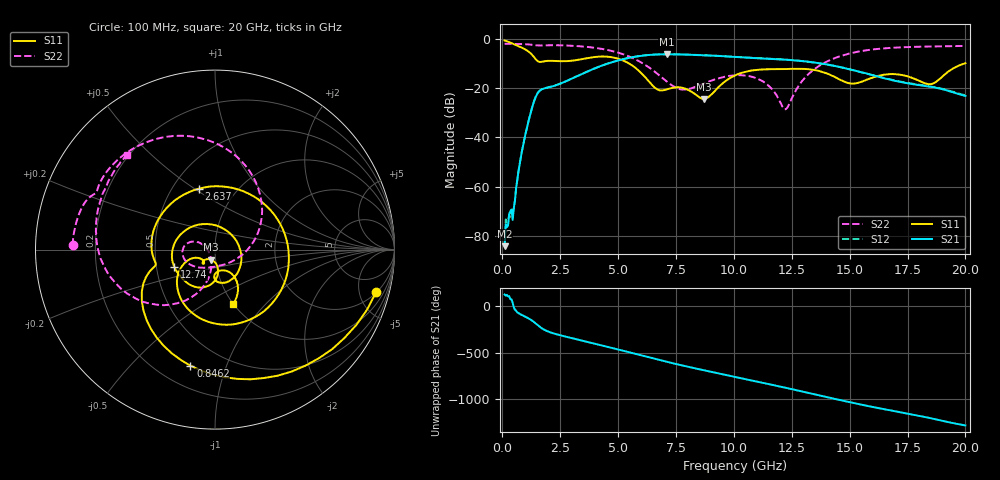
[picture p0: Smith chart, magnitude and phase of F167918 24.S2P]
!  2-Port S-parameters saved by WinCal
! VAR MeasName=S-Parameters (CALIBRATED_DATA) read from VNA (N5242A)
! VAR MeasDate=2016-11-22 10:25:54
! VAR NAME=F167918 24
! VAR FILENAME=F167918 24.S2P
! VAR DATE=2016-11-22 10:25:54
! VAR PHYS_PORTS=1,2
# Hz S DB R 50
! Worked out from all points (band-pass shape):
!   401 points, 100 MHz to 20 GHz, reference 50 ohm
!   highest |S21| = -6.24 dB at 7.115 GHz (marker M1); lowest = -84.2 dB at 100 MHz (marker M2)
!   |S21| within 3 dB of the highest: 4.827 GHz to 13.19 GHz (8.367 GHz wide, 92.9 % of centre)
!   lowest |S11| = -24.4 dB at 8.707 GHz (marker M3), VSWR 1.13, Z = 47.5 - j5.3 ohm
!   |S11| at or under -10 dB: 5.475 GHz to 19.97 GHz (14.49 GHz wide, 114 % of centre)
!   |S22| runs from -28.6 to -2.0 dB; largest |S21 - S12| = 0.0046
!   S11 on the Smith chart (normalised r, x): 100 MHz: 2.07, -7.12; 846.2 MHz: 0.33, -0.76; 2.637 GHz: 0.67, +0.52; 12.74 GHz: 0.62, -0.13; 20 GHz: 0.99, -0.68
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1e8  -0.64 -14.8  -84.24 128.8  -83.39 135.6  -2.00 178.3
4.4825e8  -1.91 -57.8  -73.55 38.5  -69.50 29.2  -2.04 172.4
8.4625e8  -3.59 -102.0  -45.74 -93.0  -45.65 -92.0  -2.12 165.5
1.493e9  -8.77 -163.2  -22.62 163.9  -22.57 163.9  -2.64 155.1
2.63725e9  -9.09 104.7  -17.69 38.5  -17.67 38.3  -2.65 136.8
3.43325e9  -8.25 25.9  -14.28 -9.3  -14.28 -9.3  -3.07 119.6
3.9805e9  -7.38 -23.0  -12.04 -42.5  -12.03 -42.4  -3.61 106.0
4.677e9  -7.38 -77.8  -9.67 -86.4  -9.62 -86.4  -4.79 86.0
5.52275e9  -10.27 -132.5  -7.63 -140.7  -7.59 -140.9  -7.35 57.0
6.7665e9  -20.82 -143.8  -6.30 139.5  -6.31 139.4  -14.71 0.8
7.11475e9  -20.48 -129.8  -6.24 118.2  -6.26 118.2  -17.41 -20.4
7.81125e9  -19.96 -133.5  -6.35 77.2  -6.34 77.3  -20.59 -75.6
8.70675e9  -24.42 -112.2  -6.63 27.1  -6.64 27.0  -18.10 -125.7
1.005e10  -14.86 -92.4  -7.31 -45.9  -7.30 -45.7  -14.82 -167.7
1.13435e10  -12.38 -125.6  -8.01 -114.3  -7.96 -114.2  -17.78 159.7
1.218925e10  -12.27 -143.4  -8.42 -159.9  -8.40 -160.1  -28.62 -162.5
1.27365e10  -12.16 -157.1  -8.82 169.4  -8.79 169.2  -20.01 -101.7
1.338325e10  -12.54 -179.8  -9.46 132.6  -9.46 132.4  -13.00 -108.3
1.507475e10  -18.16 55.6  -12.50 37.4  -12.55 37.6  -5.78 -147.5
1.67165e10  -14.34 -64.6  -16.44 -46.1  -16.41 -45.3  -3.69 178.9
1.85075e10  -18.40 -74.1  -19.47 -133.4  -19.38 -133.2  -3.11 151.8
2e10  -9.87 -71.8  -23.17 148.6  -22.95 148.8  -2.86 132.8
